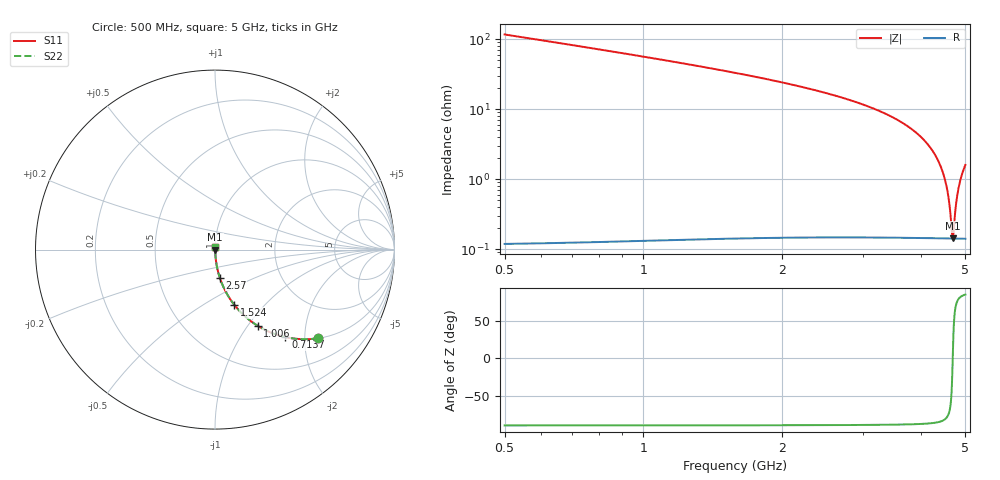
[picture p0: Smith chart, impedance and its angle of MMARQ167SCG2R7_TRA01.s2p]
! MMARQ167SCG2R7_TRA01  S-PARAMETER MODEL  ( General Type )
! Model Generated by TAIYO YUDEN Corporation (http://www.ty-top.com)
! Version 1.0
! TAIYO YUDEN Control No. 150305
! Copyright(c) 2015 TAIYO YUDEN CO.,LTD. All Rights Reserved.
! Product Description (link to TY-COMPAS)
! https://ds.yuden.co.jp/TYCOMPAS/or/detail?pn=MMARQ167SCG2R7BTRA01&u=M
! Products Name : Multilayer Ceramic Capacitors
! Characteristics :
!  Capacitance : 2.7 pF , Rated Voltage : 250V , TCC : CG / C0G
!  Case Size : 1.6 x 0.8 / 0.063 x 0.031 [mm/inch] , Thickness : 0.7 / 0.028 [mm/inch]
!  (Conditions: Temperature = 25 degC , DC Bias Current/Voltage = 0A / 0V)
! External Node Assignments :
!  1  o---| |---o  2
! GND o---------o GND
! Frequency Range : 500MHz  -  5GHz  [ 401 STEP ]
# MHz S RI R 50
! Freq[MHz].  S11 Real  S11 Imag  S21 Real  S21 Imag  S12 Real  S12 Imag  S22 Real  S22 Imag
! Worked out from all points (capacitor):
!   401 points, 500 MHz to 5 GHz, reference 50 ohm
!   read as one part in series: C = 2.71 pF near 522.5 MHz
!   lowest |Z| = 142 mohm at 4.696 GHz (marker M1)
!   series resonance near 4.693 GHz, so ESL is about 420 pH
!   S11 on the Smith chart (normalised r, x): 500 MHz: 1.00, -2.32; 713.8 MHz: 1.00, -1.61; 1.006 GHz: 1.00, -1.11; 1.524 GHz: 1.00, -0.69; 2.57 GHz: 1.00, -0.32; 5 GHz: 1.00, +0.03
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500  0.574 -0.494  0.426 0.494  0.426 0.494  0.574 -0.494
713.75  0.3925 -0.4875  0.6075 0.4875  0.6075 0.4875  0.3925 -0.4875
1006.25  0.237 -0.4241  0.763 0.4241  0.763 0.4241  0.237 -0.4241
1253.75  0.1597 -0.3648  0.8403 0.3648  0.8403 0.3648  0.1597 -0.3648
1523.75  0.1071 -0.3072  0.8929 0.3072  0.8929 0.3072  0.1071 -0.3072
2007.5  0.0552 -0.2253  0.9448 0.2253  0.9448 0.2253  0.0552 -0.2253
2570  0.0263 -0.1555  0.9737 0.1555  0.9737 0.1555  0.0263 -0.1555
2750  0.0206 -0.1371  0.9794 0.1371  0.9794 0.1371  0.0206 -0.1371
3503.75  0.0069 -0.0735  0.9931 0.0735  0.9931 0.0735  0.0069 -0.0735
3942.5  0.00335 -0.0436  0.9967 0.0436  0.9967 0.0436  0.00335 -0.0436
4257.5  0.00202 -0.0243  0.998 0.0243  0.998 0.0243  0.00202 -0.0243
4415  0.00165 -0.0153  0.9983 0.0153  0.9983 0.0153  0.00165 -0.0153
4527.5  0.0015 -0.00897  0.9985 0.00897  0.9985 0.00897  0.0015 -0.00897
4595  0.00144 -0.00528  0.9986 0.00528  0.9986 0.00528  0.00144 -0.00528
4628.75  0.00143 -0.00345  0.9986 0.00345  0.9986 0.00345  0.00143 -0.00345
4673.75  0.00141 -0.00104  0.9986 0.00104  0.9986 0.00104  0.00141 -0.00104
4696.25  0.00141 0.000159  0.9986 -0.000159  0.9986 -0.000159  0.00141 0.000159
4718.75  0.00141 0.00135  0.9986 -0.00135  0.9986 -0.00135  0.00141 0.00135
4775  0.00143 0.00431  0.9986 -0.00431  0.9986 -0.00431  0.00143 0.00431
4820  0.00145 0.00665  0.9985 -0.00665  0.9985 -0.00665  0.00145 0.00665
4898.75  0.00152 0.0107  0.9985 -0.0107  0.9985 -0.0107  0.00152 0.0107
5000  0.00165 0.0158  0.9983 -0.0158  0.9983 -0.0158  0.00165 0.0158
